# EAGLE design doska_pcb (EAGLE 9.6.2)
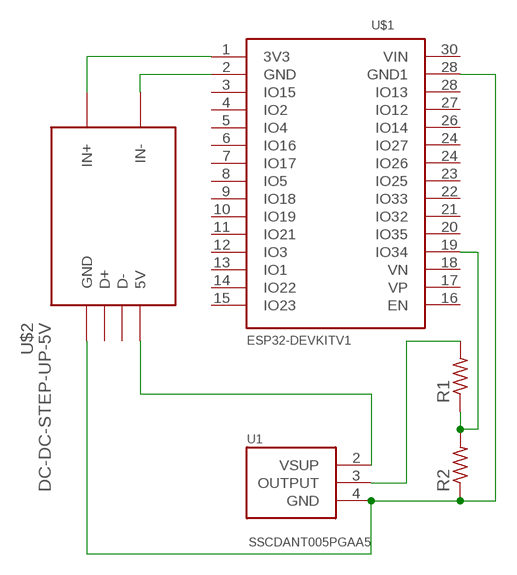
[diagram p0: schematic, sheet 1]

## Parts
R1  FLIPFLOP-RES  [0805-THM]
R2  FLIPFLOP-RES  [0805-THM]
U1  SSCDANT005PGAA5  SSCDANN150PGAA5  [XDCR_SSCDANN150PGAA5]
U$1  ESP32DEVKITV1  [ESP32-DEVKITV1]
U$2  DC-DC-STEP-UP-5V  [DC-DC-STEP-UP-5V]

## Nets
N$2: R1.2 U1.3(OUTPUT)
N$3: U$1.1(3V3) U$2.IN+
N$4: R2.1 U1.4(GND) U$1.28(GND1) U$2.GND
N$5: U1.2(VSUP) U$2.5V
N$6: U$1.2(GND) U$2.IN-
N$8: R1.1 R2.2 U$1.19(IO34)
Unconnected: U$1.3(IO15) U$1.4(IO2) U$1.5(IO4) U$1.6(IO16) U$1.7(IO17) U$1.8(IO5) U$1.9(IO18) U$1.10(IO19) U$1.11(IO21) U$1.12(IO3) U$1.13(IO1) U$1.14(IO22) U$1.15(IO23) U$1.16(EN) U$1.17(VP) U$1.18(VN) U$1.20(IO35) U$1.21(IO32) U$1.22(IO33) U$1.23(IO25) U$1.24(IO26) U$1.24(IO27) U$1.26(IO14) U$1.27(IO12) U$1.28(IO13) U$1.30(VIN) U$2.D+ U$2.D-

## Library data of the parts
R1 R2 = adafruit:FLIPFLOP-RES: Flip Flop resistor
U1 = SSCDANN150PGAA5:SSCDANN150PGAA5: Sensor; Pressure; gage; 0 psi to 150 psi; 5.0 Vdc; dry gases only Check prices; AVAILABILITY: Warning; DESCRIPTION: Pressure Sensor 150PSI (1034.21kPa) Vented Gauge Male - 0.19 (4.93mm) Tube 0.5 V ~ 4.5 V 8-DIP (0.524, 13.30mm), Top Port; MF: Honeywell Sensing; MP: SSCDANN150PGAA5; PACKAGE: DIP-8 Honeywell; PRICE: None; PURCHASE-URL: https://pricing.snapeda.com/search/part/SSCDANN150PGAA5/?ref=eda
U$1 = ESP32-DEVKITV1:ESP32DEVKITV1
U$2 = diy-modules:DC-DC-STEP-UP-5V: DC/DC Step-Up Converter

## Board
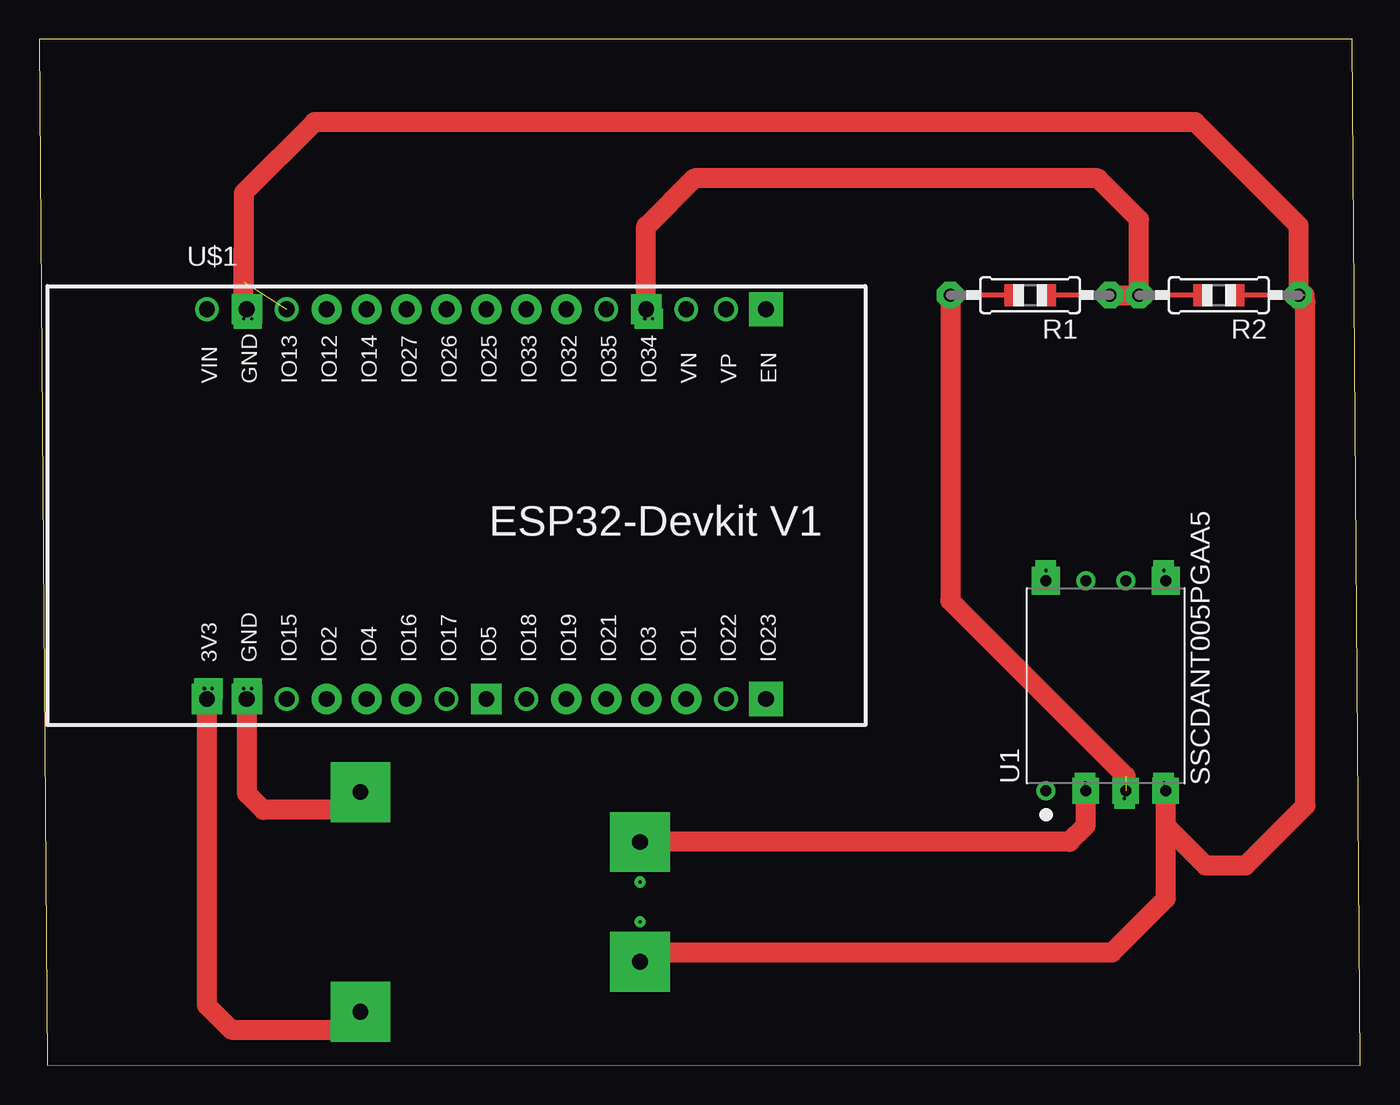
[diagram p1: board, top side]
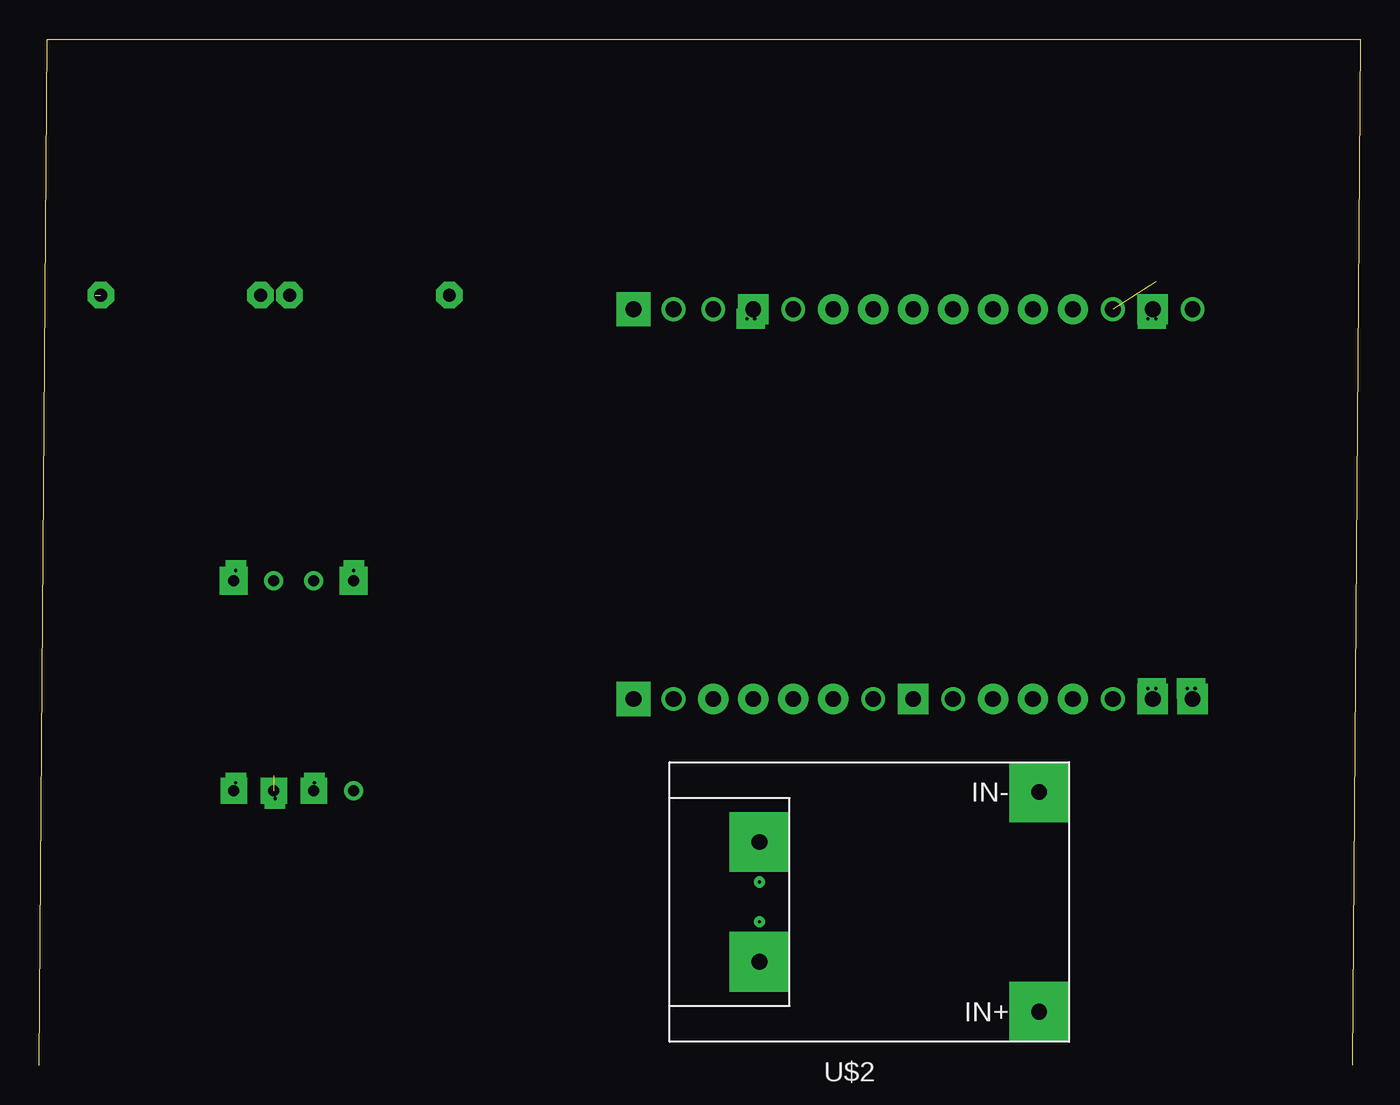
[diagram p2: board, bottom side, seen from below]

Size 83.99 x 65.22 mm. Coordinates in mm from the lower left corner, seen from the top.
Outline: 83.99,0 83.49,65.22 0,65.22 0.5,0
Copper layers (1*16): Top 0.035mm / dielectric 1.5mm / Bottom 0.035mm
Design rules "default": minimum track width 6mil, minimum drill 0.35mm, track to track 6mil, track to pad 6mil, pad to pad 6mil, via to via 6mil, smd to smd 6mil, copper to edge 40mil, drill to drill 6mil, minimum pad ring 10mil, minimum via ring 8mil, stop-mask expansion 4mil, vias tented up to drill 0mil, thermal gap 10mil

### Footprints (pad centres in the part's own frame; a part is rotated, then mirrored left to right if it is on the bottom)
0805-THM = drill 0.813 pad 1.676 octagon: 1 -5.08,0; 2 5.08,0
XDCR_SSCDANN150PGAA5 = drill 0.7 pad 1.016: 1 -6.675,3.81; 6 6.675,-1.27; 7 6.675,1.27 | drill 0.7 pad 1.676 square: 2 -6.675,1.27; 3 -6.675,-1.27; 4 -6.675,-3.81 | drill 0.7 pad 1.778 square: 5 6.675,-3.81; 8 6.675,3.81
ESP32-DEVKITV1 = drill 1 pad 1.93 square: 1 -22.87,-13.54; 2 -20.33,-13.54; 8 -5.09,-13.54; 19 5.07,11.23; 29 -20.33,11.23 | drill 1 pad 1.016: 3 -17.79,-13.54; 7 -7.63,-13.54; 9 -2.55,-13.54; 14 10.15,-13.54; 17 10.15,11.23; 18 7.61,11.23; 20 2.53,11.23; 28 -17.79,11.23; 30 -22.87,11.23 | drill 1 pad 1.93: 4 -15.25,-13.54; 5 -12.71,-13.54; 6 -10.17,-13.54; 10 -0.01,-13.54; 11 2.53,-13.54; 12 5.07,-13.54; 13 7.61,-13.54; 21 -0.01,11.23; 22 -2.55,11.23; 23 -5.09,11.23; 24 -7.63,11.23; 25 -10.17,11.23; 26 -12.71,11.23; 27 -15.25,11.23 | drill 1 pad 2.184 square: 15 12.69,-13.54; 16 12.69,11.23
DC-DC-STEP-UP-5V = drill 1 pad 3.81 square: 5V 6.985,-3.81; GND 6.985,3.81; IN+ -10.795,6.985; IN- -10.795,-6.985 | drill 0.2 pad 0.254: D+ 6.985,1.27; D- 6.985,-1.27

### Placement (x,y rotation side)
R1  63,48.96 180 top
R2  75,48.96 180 top
U1  67.81,24.13 90 top
U$1  33.52,36.83 0 top
U$2  31.21,10.39 180 bottom

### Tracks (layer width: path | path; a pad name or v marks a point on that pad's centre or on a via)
N$1
  Top 0: 0.5,0 83.99,0
N$2  (1 unrouted)
  Top 1.27: R1.2 57.92,29.54 69.06,18.4 69.08,18.4
N$3
  Top 1.27: U$1.1 10.65,3.82 12.2,2.27 19.28,2.27 U$2.IN+
N$4  (2 unrouted)
  Top 1.27: U$2.GND 38.93,6.58 39.53,7.19 68.23,7.19 71.62,10.58 U1.4 71.62,15.24 74.16,12.7 76.7,12.7 80.51,16.51 80.51,48.53 80.44,48.6 80.44,48.96 | R2.1 80.08,53.38 73.5,59.96 17.5,59.96 13,55.46 13,49.81
N$5
  Top 1.27: U1.2 66.54,15.24 65.5,14.2 U$2.5V 38.2,14.16
N$6
  Top 1.27: U$1.2 13.19,17.29 14.24,16.24 19.28,16.24 U$2.IN-
N$7  (via drill 0.2 pad 1.3)
  other vias: 66.5,17.96
N$8
  Top 0.406: 38.59,53.33 38.6,53.34
  Top 1.27: 38.6,53.34 41.64,56.38 67.31,56.38 69.92,53.77 R2.2 R1.1 | U$1.19 38.59,53.33
N$9  (via drill 0.2 pad 1.3)
  other vias: 71.5,17.96
N$10  (via drill 0.2 pad 1.3)
  other vias: 69,16.96
N$11  (via drill 0.2 pad 1.3)
  other vias: 64,31.46
N$12  (via drill 0.2 pad 1.3)
  other vias: 71.5,31.46
N$13  (via drill 0.2 pad 1.3)
  other vias: 11,23.96
N$14  (via drill 0.2 pad 1.3)
  other vias: 10.5,23.96
N$15  (via drill 0.2 pad 1.3)
  other vias: 13,23.96
N$16  (via drill 0.2 pad 1.3)
  other vias: 13.5,23.96
N$17  (via drill 0.2 pad 1.3)
  Top 1.27: v13,47.46 13,50.46 13,51.96
N$18  (via drill 0.2 pad 1.3)
  other vias: 13.5,47.46
N$19  (via drill 0.2 pad 1.3)
  other vias: 38.5,47.46
N$20  (via drill 0.2 pad 1.3)
  other vias: 39,47.46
